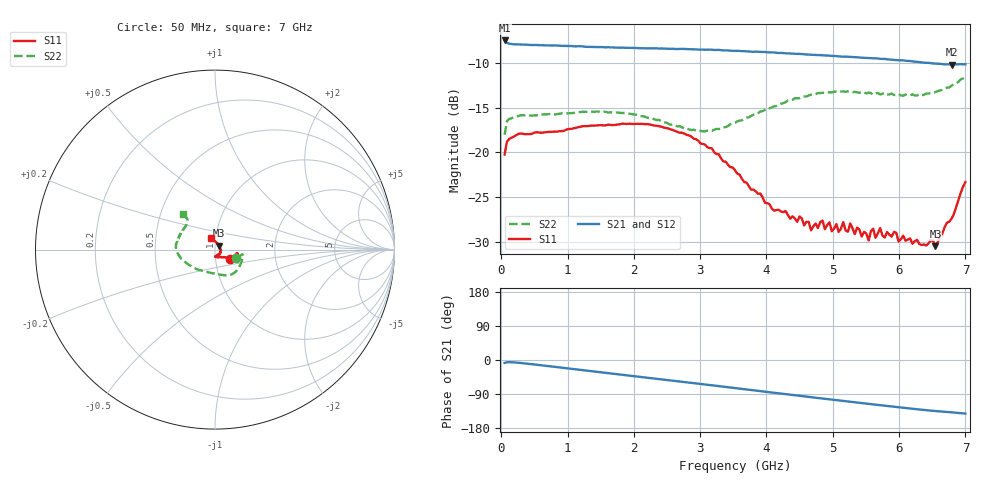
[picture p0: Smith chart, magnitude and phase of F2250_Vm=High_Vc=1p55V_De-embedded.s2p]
! Integrated Device Technology
! Corporate Headquarters
! 6024 Silver Creek Valley Road
! San Jose, CA 95138  USA
! Phone:  1-408-284-8200
! Toll Free:  1-800-223-1366
! Webpage:  http://www.idt.com/
! Timing and RF Division
! 515 Groton Road, Suite 102
! Westford, MA 01886-6024
! Device:  F2250
! Description: Voltage Variable RF Attenuator
! Frequency:  50.0 -  6000.00 MHz
! Package:  3x3 mm Thin QFN Plastic Package: 16 pin
! Ports:  2 RF, 3 DC
!  Pin  1  = GND
!  Pin  2  = NC
!  Pin  3  = RF1  = Port 1
!  Pin  4  = NC
!  Pin  5  = GND
!  Pin  6  = GND
!  Pin  7  = GND
!  Pin  8  = GND
!  Pin  9  = NC
!  Pin 10  = RF2  = Port 2
!  Pin 11  = NC
!  Pin 12  = GND
!  Pin 13  = GND
!  Pin 14  = VCNTRL
!  Pin 15  = VDD
!  Pin 16  = VMODE
! Vcntrl:  1.550 Volts
! Vmode:  +3.300 Volts
! Vdd:  +3.30  Volts
! Current:  1.328 mA
! Data:  The device was measured on a the F2250 evaluation board which has
!  individual transmission lines to the RF pins.  Data was collected
!  using a calibrated network analyzer.  The evaluation board was
!  de-embedded using a TRL calibration technique.
!  The reference plane is the edge of the package pin.
! Misc:  SN 10
!  Action Tracker AT0258
! Date Measured:  2014-11-26
! Date:  2015-10-15  MJV
! Note:
!  Integrated Device Technology supplies this data as a sample of measured
!  data at the package pin for this product.  Your particular data for this
!  product may vary.
!  Data was taken at 25 degrees C.
!  Integrated Device Technology reserves the right to change this data at anytime.
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# GHz S dB R 50
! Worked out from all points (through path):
!   201 points, 50 MHz to 7 GHz, reference 50 ohm
!   highest |S21| = -7.47 dB at 50 MHz (marker M1); lowest = -10.2 dB at 6.792 GHz (marker M2)
!   group delay of S21, straight-line fit = 56.6 ps
!   lowest |S11| = -30.5 dB at 6.548 GHz (marker M3), VSWR 1.06, Z = 52.1 + j2.25 ohm
!   |S11| at or under -10 dB: start of sweep to end of sweep
!   |S22| runs from -18.0 to -11.5 dB; largest |S21 - S12| = 0.0022
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0.05  -20.25 -31.6  -7.47 -7.8  -7.49 -7.8  -18.03 -21.5
0.08475  -18.81 -15.8  -7.75 -6.0  -7.75 -6.0  -16.52 -12.0
0.2585  -17.93 -9.5  -7.91 -7.3  -7.92 -7.3  -15.94 -12.7
1.2315  -17.07 -23.0  -8.15 -26.8  -8.18 -26.8  -15.46 -42.5
2.37825  -17.07 -24.9  -8.38 -50.0  -8.37 -50.0  -16.36 -70.9
2.969  -18.67 -25.0  -8.49 -62.3  -8.46 -62.3  -17.63 -97.9
3.525  -22.01 -34.0  -8.63 -74.1  -8.62 -74.1  -16.68 -131.2
4.11575  -26.53 -60.6  -8.82 -86.6  -8.86 -86.5  -14.84 -157.9
4.7065  -28.28 -84.2  -9.09 -98.8  -9.07 -98.8  -13.56 -174.9
4.8455  -27.65 -80.6  -9.14 -101.6  -9.11 -101.7  -13.35 -178.0
5.08875  -28.92 -78.6  -9.25 -106.6  -9.24 -106.7  -13.25 175.8
5.15825  -27.81 -78.2  -9.29 -108.0  -9.27 -108.1  -13.18 174.4
5.22775  -28.89 -79.4  -9.30 -109.5  -9.30 -109.5  -13.17 172.5
5.2625  -27.97 -75.1  -9.31 -110.1  -9.31 -110.2  -13.18 172.1
5.5405  -29.88 -62.7  -9.44 -115.8  -9.44 -115.8  -13.31 164.4
5.61  -28.55 -55.6  -9.46 -117.1  -9.46 -117.2  -13.54 163.1
5.64475  -29.58 -54.6  -9.48 -117.9  -9.48 -118.0  -13.40 161.1
5.71425  -28.47 -51.2  -9.52 -119.2  -9.52 -119.3  -13.52 160.3
5.85325  -29.22 -41.4  -9.60 -121.9  -9.61 -122.0  -13.52 155.8
6.54825  -30.51 46.4  -10.06 -134.6  -10.05 -134.8  -13.26 135.4
6.7915  -27.42 83.8  -10.16 -138.1  -10.15 -138.3  -12.53 131.7
7  -23.33 111.1  -10.14 -141.4  -10.14 -141.6  -11.52 131.5
